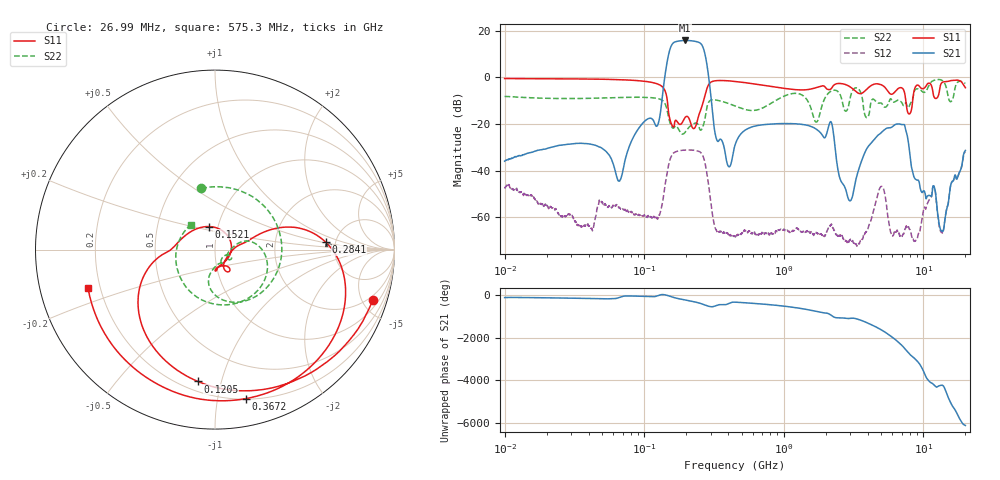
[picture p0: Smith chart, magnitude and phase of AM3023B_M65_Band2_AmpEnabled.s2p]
!Agilent Technologies,E8364B,MY43040894,A.07.50.67
!Agilent E8364B: A.07.50.67
!Date: Tuesday, October 27, 2020 10:52:28
!Correction: S11(Full 2 Port(1,2))
!S21(Full 2 Port(1,2))
!S12(Full 2 Port(1,2))
!S22(Full 2 Port(1,2))
!S2P File: Measurements: S11, S21, S12, S22:Log Frequency Sweep
# Hz S  dB  R 50
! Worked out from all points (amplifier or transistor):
!   3201 points, 10 MHz to 20 GHz, reference 50 ohm
!   highest |S21| = 15.7 dB at 197.1 MHz (marker M1)
!   |S21| within 3 dB of that: 154.5 MHz to 264.1 MHz (109.5 MHz wide, 52.3 % of centre)
!   unconditionally stable (mu >= 1): start of sweep to end of sweep
!   at 35.47 MHz: K = 2846.02, MAG = -19.8 dB, |S12| = -63.8 dB
!   at 447.2 MHz: K = 11714.51, MAG = -24.2 dB, |S12| = -68.1 dB
!   at 20 GHz: K = 208.96, MAG = -26.0 dB, |S12| = -31.8 dB
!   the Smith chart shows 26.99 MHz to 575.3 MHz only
!   S11 on the Smith chart (normalised r, x): 26.99 MHz: 1.60, -6.01; 120.5 MHz: 0.26, -0.84; 152.1 MHz: 0.90, +0.24; 284.1 MHz: 4.16, +0.56; 367.2 MHz: 0.20, -1.21; 575.3 MHz: 0.15, -0.14
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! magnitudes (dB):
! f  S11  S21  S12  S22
! 10 MHz  -0.6  -36.0  -47.7  -8.2
! 26.99 MHz  -0.7  -28.9  -59.4  -9.1
! 35.55 MHz  -0.8  -28.3  -63.9  -9.1
! 66.24 MHz  -1.1  -44.5  -56.0  -8.7
! 120.5 MHz  -2.6  -20.6  -60.1  -9.0
! 126.1 MHz  -3.0  -19.9  -59.8  -9.2
! 152.1 MHz  -17.5  11.5  -35.8  -19.0
! 197.1 MHz  -17.1  15.7  -31.2  -23.5
! 284.1 MHz  -4.2  3.8  -42.9  -11.9
! 367.2 MHz  -1.4  -28.4  -66.9  -10.5
! 447.2 MHz  -1.8  -29.1  -68.1  -12.3
! 575.3 MHz  -2.6  -21.5  -66.4  -14.2
! 1.59 GHz  -5.0  -21.2  -66.8  -14.6
! 2.186 GHz  -4.9  -19.2  -63.1  -5.9
! 2.984 GHz  -4.1  -52.9  -69.7  -9.1
! 4.972 GHz  -3.2  -23.9  -46.8  -11.0
! 5.639 GHz  -6.5  -21.7  -61.5  -11.0
! 7.305 GHz  -6.3  -20.3  -66.2  -12.0
! 8.751 GHz  -4.2  -43.6  -70.2  -5.3
! 11.83 GHz  -7.9  -46.5  -46.5  -1.4
! 13.52 GHz  -2.4  -65.9  -66.2  -1.3
! 20 GHz  -4.5  -31.3  -31.8  -2.6
